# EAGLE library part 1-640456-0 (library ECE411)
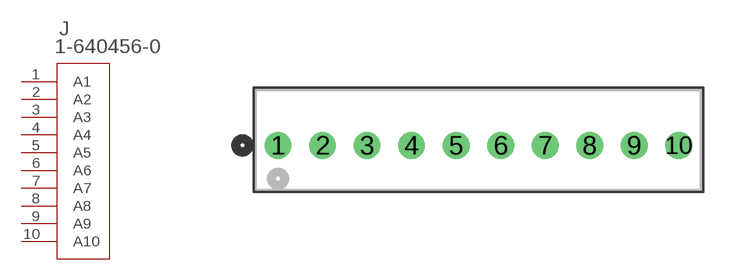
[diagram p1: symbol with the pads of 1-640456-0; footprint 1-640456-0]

Designator prefix J

## 1-640456-0 (MANUFACTURER_PART_NUMBER: 16404560; VENDOR: TE Connectivity)  [1-640456-0]
1  A1  pas
2  A2  pas
3  A3  pas
4  A4  pas
5  A5  pas
6  A6  pas
7  A7  pas
8  A8  pas
9  A9  pas
10  A10  pas

## Footprint 1-640456-0 (pad centres in mm)
drill 1.016 pad 1.524: 1 -22.86,0; 2 -20.32,0; 3 -17.78,0; 4 -15.24,0; 5 -12.7,0; 6 -10.16,0; 7 -7.62,0; 8 -5.08,0; 9 -2.54,0; 10 0,0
